PROGRAM Communication
VAR
	// Tc2_DALI	
	fbKL6821CommunicationTc2		:	Tc2_DALI.FB_KL6821Communication;
	
	// Tc3_DALI
	fbKL6821CommunicationTc3		:	Tc3_DALI.FB_KL6821Communication;	
END_VAR

// Tc2_DALI
fbKL6821CommunicationTc2(	stInData := GVL.stKL6821InDataTc2,
							stOutData := GVL.stKL6821OutDataTc2,
							stCommandBuffer := GVL.stCommandBufferKL6821);

// Tc3_DALI			 
fbKL6821CommunicationTc3(	stInData := GVL.stKL6821InDataTc3,
							stOutData := GVL.stKL6821OutDataTc3);

END_PROGRAM
